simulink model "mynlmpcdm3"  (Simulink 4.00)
settings: Solver=ode45  SolverMode=SingleTasking  StartTime=0.0  StopTime=30*100  FixedStep=[]  MaxStep=1  RelTol=1e-3  AbsTol=1e-3
PreLoadFcn:
  | demo2dat
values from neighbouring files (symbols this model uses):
  d0 = []    [demo1dat.m]    (also in demo2dat.m = 0; essai1dat.m)
  dmodel = []    [demo1dat.m]    (also in essai1dat.m; essai2dat.m; mynlcmpc.m = modelpd(:,nu+1:nund); mynlcmpc2.m = modelpd(:,nu+1:nund))
  m = 4    [demo1dat.m]    (also in demo2dat.m = 3; essai1dat.m; essai2dat.m = 6; mynlcmpc.m = mp(1:max(size(mp))-1))
  model = tfd2step(1.6,delt,1,g)    [essai2dat.m]    (also in mynlcmpc.m = modelpd(:,1:nu); mynlcmpc2.m = modelpd(:,1:nu); mynlcmpc3.m = modelpd(:,1:nu); scrtp1.m = tfd2step(tfinal,Ts,1,g))
  p = 10    [demo1dat.m]    (also in demo2dat.m; essai1dat.m; essai2dat.m; mynlcmpc.m = mp(max(size(mp))))
  r = [68.3 2]    [demo1dat.m]    (also in demo2dat.m = [0 0 0]; essai1dat.m; essai2dat.m = 10; mynlcmpc.m = zeros(1,ny))
  tfilter = [0 1]    [demo1dat.m]    (also in demo2dat.m = []; essai1dat.m)
  u0 = [100 1]    [demo1dat.m]    (also in demo2dat.m = [0 0]; essai1dat.m; pmnonl.m = zeros(3,1))
  u_lim = [100 1 200 3 200 200]    [demo1dat.m]    (also in demo2dat.m = [-10*[1 1] 10*[1 1] 2*[1 1]]; essai1dat.m)
  uwt = [0 0]    [demo1dat.m]    (also in demo2dat.m = 0.6*[1 1]; essai1dat.m; essai2dat.m = 1; mynlcmpc.m = ryuwt(:,2*ny+1:2*ny+nu))
  y_lim = [-inf -inf inf inf]    [demo1dat.m]    (also in demo2dat.m = [-inf -inf -inf inf inf inf]; essai1dat.m)
  ywt = [1 1]    [demo1dat.m]    (also in demo2dat.m = [0.2,0,1]; essai1dat.m; essai2dat.m = 1; mynlcmpc.m = ryuwt(:,ny+1:2*ny))

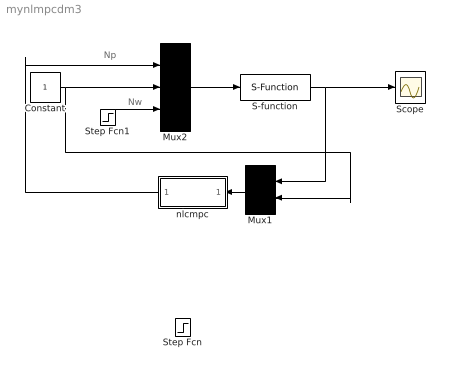
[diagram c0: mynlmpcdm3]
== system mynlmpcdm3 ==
  note: Nw
  note: Np
  Constant : Constant  Value=1
  Mux1 : Mux  Orientation=left  Inputs=[3 1]
  Mux2 : Mux  Inputs=[2 1 1]
  S-function : S-Function  FunctionName=papmach  PortCounts=[]  SFunctionModules=''
  Scope : Scope
  Step Fcn : Step  Time=0  Before=0  After=1  SampleTime=0
  Step Fcn1 : Step  Time=0  Before=0  After=0  SampleTime=0
  nlcmpc : Subsystem  Orientation=left  AncestorBlock=nlmpclib/nlcmpc  mask(myCMPC-SIMULINK){modelpd=[model dmodel], ryuwt=[r ywt uwt], mp=[m p], yulim=[y_lim u_lim], tfilter=tfilter, ud0=[u0 d0]}
      mask help: Masked MATLAB function block calls nlcmpc, links CMPC and SIMULINK.
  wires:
  S-function/1 -> Mux1/1, Scope/1
  Constant/1 -> Mux2/2, Mux1/2
  Step Fcn1/1 -> Mux2/3
  Mux2/1 -> S-function/1
  nlcmpc/1(Out1) -> Mux2/1
  Mux1/1 -> nlcmpc/1(In1)

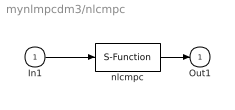
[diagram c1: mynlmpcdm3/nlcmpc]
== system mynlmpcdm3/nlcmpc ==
  In1 : Inport  Port=1  LatchInput=off
  nlcmpc : S-Function  FunctionName=mynlcmpc  Parameters=modelpd,mp,tfilter,ryuwt,ud0,yulim  PortCounts=[]  SFunctionModules=''
  Out1 : Outport  Port=1  InitialOutput=0
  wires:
  In1/1 -> nlcmpc/1
  nlcmpc/1 -> Out1/1
